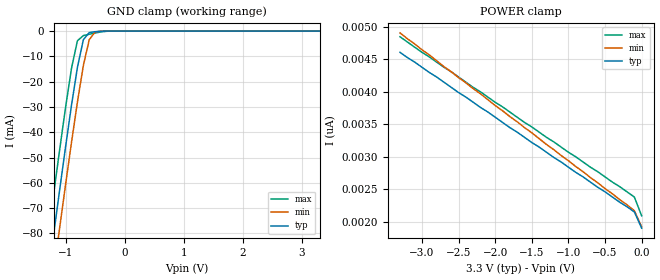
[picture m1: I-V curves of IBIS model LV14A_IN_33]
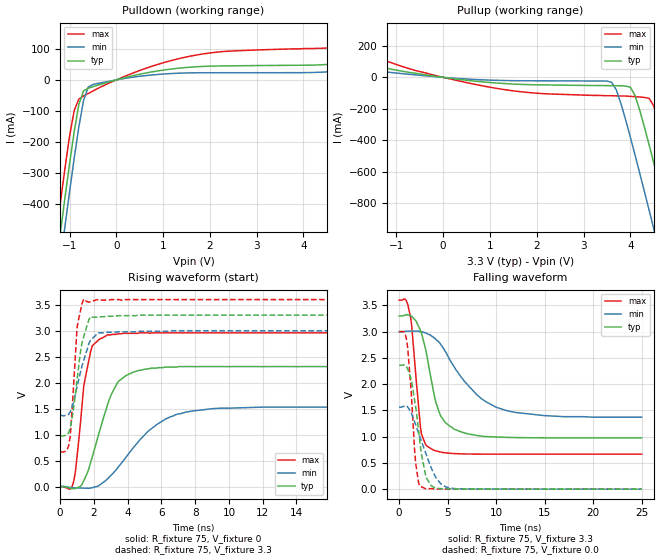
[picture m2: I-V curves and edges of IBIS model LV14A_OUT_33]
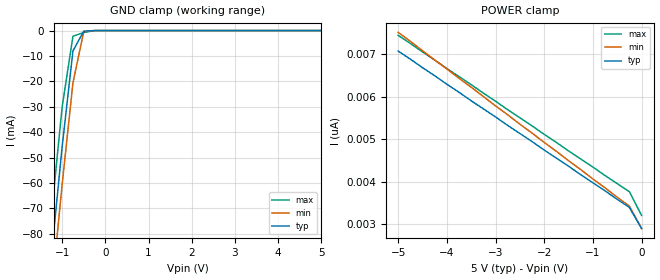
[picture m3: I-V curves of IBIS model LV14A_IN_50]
| TEXAS INSTRUMENTS INCORPORATED
| Standard Linear and Logic Group
| IBIS Model of SN74LV14A
| HEX SCHMITT-TRIGGER INVERTER
| SOIC 14-pin (D), SOP 14-pin (NS), SSOP 14-pin (DB), TSSOP 14-pin (PW)
| and TVSOP 14-pin (DGV) Package
[IBIS Ver]   3.2
[Comment Char]  |_char
[File Name]   lv14a.ibs
[File Rev]   2.0 H_die
[Date]   May 29, 2000
[Source]   Data created from HSPICE simulations at TI-SLL.
[Notes]   The following is an IBIS list for the LV14A.
|   Please contact sllibis@ti.com with questions and
|   comments concerning SLL IBIS models.
|   The warning about AC Rising Endpoint might be reported,
|   but it is due to HSPICE issue and negligible.
[Disclaimer] Property of Texas Instruments Incorporated.  Unauthorized
   reproduction and/or distribution is strictly prohibited.
   This product is protected under copyright law.
   Created 2000, (C) Copyright 2000, Texas Instruments Inc.,
   All Rights Reserved.
   UNLESS THERE IS A SIGNED, WRITTEN AGREEMENT TO THE
   CONTRARY, TEXAS INSTRUMENTS () IS PROVIDING THE IBIS
   MODELS  AND WITHOUT ANY WARRANTY, EXPRESSED OR
   IMPLIED.  TI assumes no liability for:
   1) the accuracy of the IBIS models provided to your
   company;
   2) the proper functioning of these IBIS Models in your
   design or for any resulting applications; or
   3) infringement of patents, copyrights or intellectual
   property rights resulting from your use of these IBIS
   models.
   TI provides IBIS Models as a service to our customers.
   You and your company shall not distribute, sell or give
   these models to anyone else without prior written
   permission from TI.
   TI reserves the right to make changes to our products or
   to discontinue any semiconductor product or service
   without notice, and advises our customers to obtain the
   latest version of relevant information to verify, before
   placing orders, that the information being relied on is
   current.
   Please be aware that your receipt and use of the IBIS
   information provided shall serve as acceptance of these
   terms and conditions.  If you do not accept these terms,
   you should return or destroy the IBIS models and any
   other accompanying information immediately.
|   Component LV14A_D
[Component]   LV14A_D
[Manufacturer]  Texas Instruments, Inc.
[Package]
|   typ   min   max
R_pkg   0.031   0.028   0.034
L_pkg   3.109nH   2.462nH   3.889nH
C_pkg   0.473pF   0.363pF   0.628pF
[Pin]   signal_name   model_name   R_pin   L_pin   C_pin
1   1A   LV14A_IN   0.033   3.854nH   0.622pF
2   1Y   LV14A_OUT   0.032   3.188nH   0.473pF
3   2A   LV14A_IN   0.028   2.462nH   0.377pF
4   2Y   LV14A_OUT   0.031   2.596nH   0.363pF
5   3A   LV14A_IN   0.028   2.521nH   0.372pF
6   3Y   LV14A_OUT   0.034   3.250nH   0.476pF
7   GND   GND   0.034   3.889nH   0.628pF
8   4Y   LV14A_OUT   0.034   3.889nH   0.628pF
9   4A   LV14A_IN   0.034   3.250nH   0.476pF
10   5Y   LV14A_OUT   0.028   2.521nH   0.372pF
11   5A   LV14A_IN   0.031   2.596nH   0.364pF
12   6Y   LV14A_OUT   0.028   2.462nH   0.377pF
13   6A   LV14A_IN   0.032   3.188nH   0.473pF
14   VCC   POWER   0.033   3.854nH   0.622pF
|   Component LV14A_NS
[Component]   LV14A_NS
[Manufacturer]  Texas Instruments, Inc.
[Package]
|   typ   min   max
R_pkg   0.045   0.039   0.054
L_pkg   3.796nH   2.561nH   4.952nH
C_pkg   0.528pF   0.288pF   0.710pF
[Pin]   signal_name   model_name   R_pin   L_pin   C_pin
1   1A   LV14A_IN   0.047   4.867nH   0.706pF
2   1Y   LV14A_OUT   0.051   4.083nH   0.592pF
3   2A   LV14A_IN   0.041   2.915nH   0.376pF
4   2Y   LV14A_OUT   0.039   2.561nH   0.288pF
5   3A   LV14A_IN   0.041   3.101nH   0.430pF
6   3Y   LV14A_OUT   0.047   4.047nH   0.589pF
7   GND   GND   0.051   4.909nH   0.700pF
8   4Y   LV14A_OUT   0.045   4.784nH   0.694pF
9   4A   LV14A_IN   0.054   4.176nH   0.597pF
10   5Y   LV14A_OUT   0.039   3.287nH   0.449pF
11   5A   LV14A_IN   0.039   2.586nH   0.294pF
12   6Y   LV14A_OUT   0.040   2.802nH   0.371pF
13   6A   LV14A_IN   0.049   4.080nH   0.593pF
14   VCC   POWER   0.052   4.952nH   0.710pF
|   Component LV14A_DB
[Component]   LV14A_DB
[Manufacturer]  Texas Instruments, Inc.
[Package]
|   typ   min   max
R_pkg   0.044   0.041   0.046
L_pkg   3.551nH   3.258nH   3.927nH
C_pkg   0.402pF   0.360pF   0.421pF
[Pin]   signal_name   model_name   R_pin   L_pin   C_pin
1   1A   LV14A_IN   0.046   3.927nH   0.408pF
2   1Y   LV14A_OUT   0.044   3.587nH   0.421pF
3   2A   LV14A_IN   0.041   3.289nH   0.398pF
4   2Y   LV14A_OUT   0.042   3.258nH   0.360pF
5   3A   LV14A_IN   0.041   3.286nH   0.403pF
6   3Y   LV14A_OUT   0.044   3.586nH   0.421pF
7   GND   GND   0.046   3.927nH   0.408pF
8   4Y   LV14A_OUT   0.046   3.927nH   0.408pF
9   4A   LV14A_IN   0.044   3.586nH   0.421pF
10   5Y   LV14A_OUT   0.041   3.286nH   0.403pF
11   5A   LV14A_IN   0.043   3.258nH   0.360pF
12   6Y   LV14A_OUT   0.041   3.289nH   0.398pF
13   6A   LV14A_IN   0.044   3.587nH   0.421pF
14   VCC   POWER   0.046   3.927nH   0.408pF
|   Component LV14A_PW
[Component]   LV14A_PW
[Manufacturer]  Texas Instruments, Inc.
[Package]
|   typ   min   max
R_pkg   0.032   0.029   0.035
L_pkg   2.378nH   2.170nH   2.680nH
C_pkg   0.314pF   0.270pF   0.335pF
[Pin]   signal_name   model_name   R_pin   L_pin   C_pin
1   1A   LV14A_IN   0.033   2.618nH   0.330pF
2   1Y   LV14A_OUT   0.031   2.313nH   0.317pF
3   2A   LV14A_IN   0.030   2.310nH   0.314pF
4   2Y   LV14A_OUT   0.031   2.173nH   0.272pF
5   3A   LV14A_IN   0.030   2.204nH   0.309pF
6   3Y   LV14A_OUT   0.032   2.315nH   0.317pF
7   GND   GND   0.035   2.680nH   0.335pF
8   4Y   LV14A_OUT   0.033   2.640nH   0.333pF
9   4A   LV14A_IN   0.034   2.347nH   0.319pF
10   5Y   LV14A_OUT   0.029   2.277nH   0.313pF
11   5A   LV14A_IN   0.031   2.170nH   0.270pF
12   6Y   LV14A_OUT   0.031   2.244nH   0.311pF
13   6A   LV14A_IN   0.033   2.343nH   0.321pF
14   VCC   POWER   0.035   2.657nH   0.332pF
|   Component LV14A_DGV
[Component]   LV14A_DGV
[Manufacturer]  Texas Instruments, Inc.
[Package]
|   typ   min   max
R_pkg   0.035   0.020   0.045
L_pkg   2.499nH   2.077nH   2.966nH
C_pkg   0.361pF   0.305pF   0.416pF
[Pin]   signal_name   model_name   R_pin   L_pin   C_pin
1   1A   LV14A_IN   0.027   2.717nH   0.373pF
2   1Y   LV14A_OUT   0.037   2.434nH   0.398pF
3   2A   LV14A_IN   0.034   2.200nH   0.316pF
4   2Y   LV14A_OUT   0.020   2.077nH   0.309pF
5   3A   LV14A_IN   0.030   2.147nH   0.305pF
6   3Y   LV14A_OUT   0.042   2.580nH   0.408pF
7   GND   GND   0.039   2.921nH   0.385pF
8   4Y   LV14A_OUT   0.033   2.841nH   0.380pF
9   4A   LV14A_IN   0.042   2.611nH   0.410pF
10   5Y   LV14A_OUT   0.038   2.331nH   0.329pF
11   5A   LV14A_IN   0.026   2.223nH   0.319pF
12   6Y   LV14A_OUT   0.034   2.259nH   0.313pF
13   6A   LV14A_IN   0.045   2.681nH   0.416pF
14   VCC   POWER   0.042   2.966nH   0.386pF
[Model Selector]   LV14A_IN
LV14A_IN_33   3.3-V Vcc Input Model
LV14A_IN_50   5.0-V Vcc Input Model
[Model Selector]   LV14A_OUT
LV14A_OUT_33   3.3-V Vcc Output Model
LV14A_OUT_50   5.0-V Vcc Output Model
| Models and submodels in the file (4): LV14A_IN_33 (Input), LV14A_OUT_33 (Output), LV14A_IN_50 (Input), LV14A_OUT_50 (Output)
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|   Model LV14A_IN_33
[Model]   LV14A_IN_33
Model_type  Input
Polarity   Inverting
Vinl = 0.99
Vinh = 2.31
| variable   typ   min   max
C_comp   1.26pf   0.94pf   1.58pf
[Temperature Range]   25   85   -40
[Voltage Range]   3.3   3.0   3.6
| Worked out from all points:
|   GND clamp passes 1 mA (typ) near -0.61 V on its own axis
[GND Clamp]
|   Voltage   I(typ)   I(min)   I(max)
-3.3V     -460mA     -475mA     -445mA
-1.3V     -97.5mA    -113mA     -81.5mA
-1.2V     -79.9mA    -95mA      -63.9mA
-1.1V     -62.6mA    -77.6mA    -46.7mA
-1V       -45.6mA    -60.5mA    -30mA
-900mV    -29.2mA    -43.9mA    -14.6mA
-800mV    -14.3mA    -28mA      -3.81mA
-700mV    -3.42mA    -13.6mA    -1.78mA
-600mV    -581uA     -3.4mA     -1.25mA
-500mV    -233uA     -353uA     -759uA
-400mV    -58.1uA    -21.9uA    -324uA
3.3V      1.9nA      2.34nA     1.69nA
[POWER Clamp]
|   Voltage   I(typ)   I(min)   I(max)
-3.3V     4.61nA     4.91nA     4.85nA
-3V       4.38nA     4.65nA     4.61nA
-100mV    2.15nA     2.17nA     2.38nA
0V        1.9nA      1.92nA     2.09nA
|   Model LV14A_OUT_33
[Model]   LV14A_OUT_33
Model_type  Output
Polarity   Non-Inverting
Vmeas = 1.65v
Cref = 15pf
| variable   typ   min   max
C_comp   4.62pf   3.47pf   5.77pf
[Temperature Range]   25   85   -40
[Voltage Range]   3.3   3.0   3.6
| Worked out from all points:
|   slope of the pulldown table from 0 to 0.495 V, typ, clamps not added: 27.3 ohm
|   slope of the pullup table from 0 to 0.495 V, typ, clamps not added: 27.2 ohm
|   rising waveform, R_fixture 75, V_fixture 0: 20-80 % time 1.34ns typ, 2.6ns min, 656ps max; typ from 0 V to 2.31 V
|   falling waveform, R_fixture 75, V_fixture 3.3: 20-80 % time 1.69ns typ, 4.11ns min, 821ps max; typ from 3.3 V to 0.976 V
|   rising waveform, R_fixture 75, V_fixture 3.3: 20-80 % time 586ps typ, 788ps min, 331ps max; typ from 0.976 V to 3.3 V
|   falling waveform, R_fixture 75, V_fixture 0.0: 20-80 % time 1.08ns typ, 1.88ns min, 646ps max; typ from 2.36 V to 0 V
[Pulldown]
|   Voltage   I(typ)   I(min)   I(max)
-3.3V     -3.04A     -3.13A     -2.95A
-1.3V     -615mA     -707mA     -518mA
-1.2V     -498mA     -591mA     -401mA
-1.1V     -383mA     -475mA     -288mA
-900mV    -167mA     -253mA     -98.6mA
-800mV    -79.1mA    -151mA     -61.7mA
-700mV    -35.5mA    -66.4mA    -51.9mA
-600mV    -26.8mA    -23.2mA    -43.9mA
-500mV    -22mA      -14.7mA    -35.8mA
1.6V      41.2mA     22.8mA     77.1mA
4.7V      52.1mA     27.5mA     106mA
6.6V      86.8mA     47.3mA     166mA
[Pullup]
|   Voltage   I(typ)   I(min)   I(max)
-3.3V     166mA      91.1mA     311mA
600mV     -21.6mA    -12.3mA    -39.7mA
3.6V      -52.9mA    -31.5mA    -117mA
3.8V      -54.2mA    -168mA     -119mA
4V        -62.6mA    -381mA     -121mA
4.1V      -115mA     -494mA     -123mA
4.4V      -429mA     -845mA     -133mA
4.5V      -544mA     -964mA     -182mA
4.8V      -899mA     -1.32A     -505mA
4.9V      -1.02A     -1.44A     -622mA
5.2V      -1.38A     -1.81A     -981mA
6.6V      -3.09A     -3.52A     -2.69A
[Ramp]
| variable   typ   min   max
dV/dt_r   1.40E+00/1.34E-09   9.37E-01/2.69E-09   1.78E+00/5.93E-10
dV/dt_f   1.41E+00/1.66E-09   9.88E-01/4.15E-09   1.77E+00/7.96E-10
R_load = 75
[Rising Waveform]
R_fixture = 75
V_fixture = 0
|   Time   V(typ)   V(min)   V(max)
0s        0V         0V         0V
800ps     -40.6mV    -22.2mV    94.5mV
1.1ns     -9.32mV    -26.2mV    879mV
1.4ns     115mV      -29.5mV    1.94V
1.8ns     457mV      -28.9mV    2.59V
2.8ns     1.57V      146mV      2.92V
3.9ns     2.14V      565mV      2.95V
5.7ns     2.28V      1.19V      2.96V
7.5ns     2.31V      1.44V      2.96V
25ns      2.31V      1.53V      2.96V
[Falling Waveform]
R_fixture = 75
V_fixture = 3.3
V_fixture_min = 3.0
V_fixture_max = 3.6
|   Time   V(typ)   V(min)   V(max)
0s        3.3V       3V         3.6V
700ps     3.32V      3.01V      3.6V
1.2ns     3.3V       3.01V      3.25V
2.2ns     3.02V      3V         1.17V
3.1ns     2.29V      2.94V      792mV
3.8ns     1.64V      2.85V      729mV
4.3ns     1.39V      2.75V      706mV
6.5ns     1.08V      2.11V      672mV
11ns      987mV      1.5V       666mV
25ns      976mV      1.37V      666mV
[Rising Waveform]
R_fixture = 75
V_fixture = 3.3
V_fixture_min = 3.0
V_fixture_max = 3.6
|   Time   V(typ)   V(min)   V(max)
0s        976mV      1.37V      666mV
400ps     995mV      1.37V      707mV
600ps     1.13V      1.44V      969mV
800ps     1.52V      1.64V      1.96V
1ns       2.05V      1.92V      3.06V
1.2ns     2.59V      2.2V       3.38V
1.4ns     2.89V      2.43V      3.61V
1.8ns     3.27V      2.82V      3.56V
2.7ns     3.28V      2.97V      3.59V
25ns      3.3V       3V         3.6V
[Falling Waveform]
R_fixture = 75
V_fixture = 0.0
|   Time   V(typ)   V(min)   V(max)
0s        2.36V      1.56V      3V
500ps     2.37V      1.58V      3V
800ps     2.32V      1.58V      2.81V
1.2ns     2.12V      1.47V      1.96V
1.7ns     1.57V      1.23V      500mV
2.1ns     959mV      1.02V      60.8mV
2.8ns     220mV      656mV      1.25mV
3.8ns     17.3mV     217mV      -544uV
5.8ns     2.92mV     10.1mV     -368uV
25ns      13.9uV     6.46uV     11.9uV
|   Model LV14A_IN_50
[Model]   LV14A_IN_50
Model_type  Input
Polarity   Inverting
Vinl = 1.5
Vinh = 3.5
| variable   typ   min   max
C_comp   1.26pf   0.94pf   1.58pf
[Temperature Range]   25   85   -40
[Voltage Range]   5.0   4.5   5.5
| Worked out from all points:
|   GND clamp passes 1 mA (typ) near -0.52 V on its own axis
[GND Clamp]
|   Voltage   I(typ)   I(min)   I(max)
-5V       -773mA     -786mA     -758mA
-1.5V     -133mA     -148mA     -117mA
-1.25V    -88.7mA    -104mA     -72.7mA
-1V       -45.6mA    -60.5mA    -30mA
-750mV    -7.99mA    -20.5mA    -2.23mA
-500mV    -233uA     -353uA     -759uA
-250mV    -2.63nA    -182nA     -26.9uA
5V        2.9nA      3.64nA     2.54nA
[POWER Clamp]
|   Voltage   I(typ)   I(min)   I(max)
-5V       7.08nA     7.52nA     7.45nA
-1.5V     4.37nA     4.5nA      4.73nA
-250mV    3.4nA      3.43nA     3.77nA
0V        2.9nA      2.91nA     3.21nA
